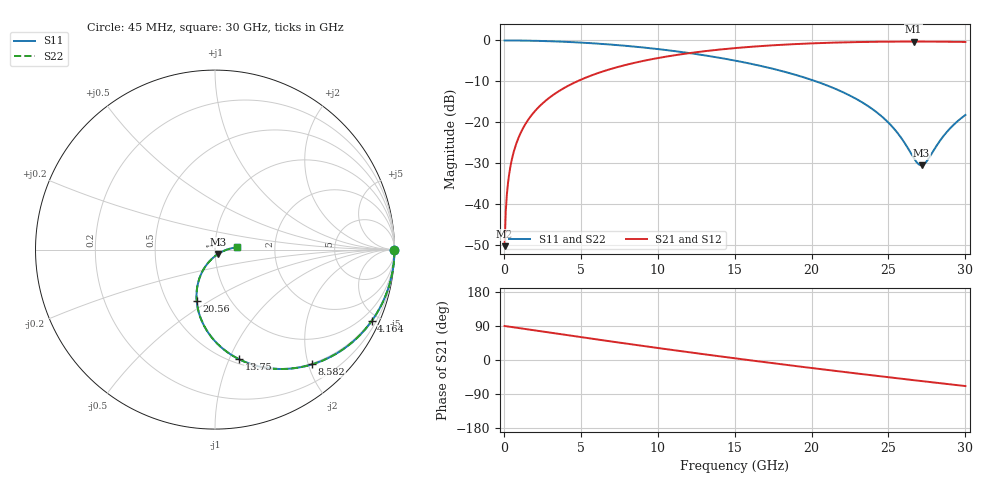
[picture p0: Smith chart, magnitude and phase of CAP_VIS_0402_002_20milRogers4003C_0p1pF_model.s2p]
! S-parameter model data by Modelithics Inc.  support@modelithics.com  813-866-6335  Tampa FL USA
! S-Parameter data specifications:
! Substrate: 20-mil Rogers 4003C, substrate thickness, H=0.508mm, Dielectric constant, Er=3.75
! PCB Mounting Pad Footprint: Pad width, PadW=0.50mm , Pad length, PadL=0.50mm , Pad gap, PadG (edge-to-edge)=0.40mm , Reference planes=1.4mm apart
! Created Wed Nov 18 11:57:18 2015
# hz S ma R 50
! 2 Port Network Data from SP1.SP block
! freq  magS11  angS11  magS21  angS21  magS12  angS12  magS22  angS22
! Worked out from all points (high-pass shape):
!   401 points, 45 MHz to 30 GHz, reference 50 ohm
!   highest |S21| = -0.27 dB at 26.63 GHz (marker M1); lowest = -50.2 dB at 45 MHz (marker M2)
!   |S21| within 3 dB of the highest: 11.72 GHz to end of sweep
!   lowest |S11| = -30.5 dB at 27.15 GHz (marker M3), VSWR 1.06, Z = 51.7 - j2.54 ohm
!   |S11| at or under -10 dB: 20.3 GHz to end of sweep
!   |S22| runs from -30.5 to 0.0 dB; largest |S21 - S12| = 0
!   S11 on the Smith chart (normalised r, x): 45 MHz: open; 4.164 GHz: 0.45, -4.55; 8.582 GHz: 0.48, -2.06; 13.75 GHz: 0.54, -1.09; 20.56 GHz: 0.70, -0.44; 30 GHz: 1.28, +0.03
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4.5e7  1 -0.3  0.003078 89.7  0.003078 89.7  1 -0.3
2.696625e8  0.9998 -1.6  0.01844 88.4  0.01844 88.4  0.9998 -1.6
4.194375e8  0.9996 -2.5  0.02868 87.5  0.02868 87.5  0.9996 -2.5
6.441e8  0.999 -3.8  0.04403 86.2  0.04403 86.2  0.999 -3.8
1.018538e9  0.9975 -6.0  0.06957 83.9  0.06957 83.9  0.9975 -6.0
1.54275e9  0.9943 -9.1  0.1052 80.8  0.1052 80.8  0.9943 -9.1
2.216738e9  0.9883 -13.1  0.1507 76.8  0.1507 76.8  0.9883 -13.1
4.163812e9  0.9594 -24.5  0.2788 65.3  0.2788 65.3  0.9594 -24.5
5.062462e9  0.9405 -29.8  0.3356 60.0  0.3356 60.0  0.9405 -29.8
8.582175e9  0.8375 -49.8  0.5382 39.7  0.5382 39.7  0.8375 -49.8
1.007992e10  0.7821 -58.0  0.613 31.3  0.613 31.3  0.7821 -58.0
1.374941e10  0.6264 -77.5  0.7647 11.2  0.7647 11.2  0.6264 -77.5
1.50225e10  0.5678 -84.0  0.8067 4.4  0.8067 4.4  0.5678 -84.0
2.003996e10  0.3285 -107.5  0.9218 -21.3  0.9218 -21.3  0.3285 -107.5
2.056418e10  0.3034 -109.6  0.9296 -23.9  0.9296 -23.9  0.3034 -109.6
2.318524e10  0.1803 -118.6  0.9573 -36.8  0.9573 -36.8  0.1803 -118.6
2.505742e10  0.09659 -119.0  0.967 -45.8  0.967 -45.8  0.09659 -119.0
2.663006e10  0.03708 -90.8  0.9694 -53.2  0.9694 -53.2  0.03708 -90.8
2.715428e10  0.02991 -55.3  0.9691 -55.6  0.9691 -55.6  0.02991 -55.3
2.752871e10  0.03436 -29.2  0.9686 -57.4  0.9686 -57.4  0.03436 -29.2
2.887669e10  0.07949 3.0  0.9647 -63.6  0.9647 -63.6  0.07949 3.0
3e10  0.1231 5.8  0.9591 -68.8  0.9591 -68.8  0.1231 5.8
